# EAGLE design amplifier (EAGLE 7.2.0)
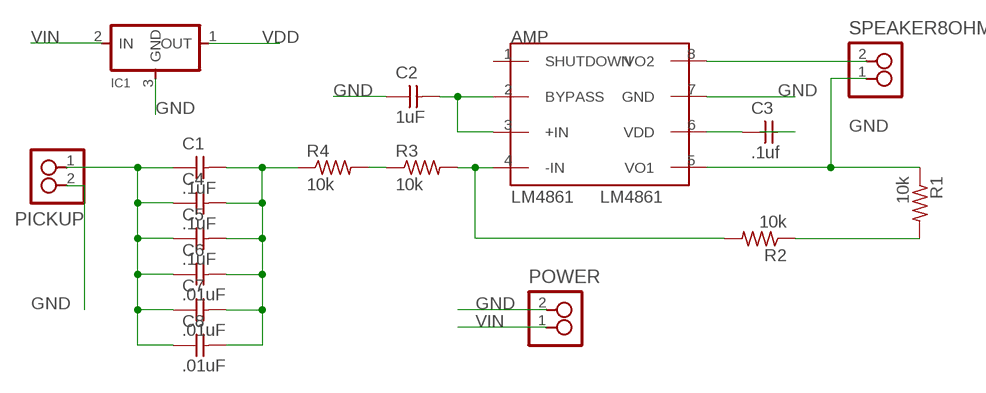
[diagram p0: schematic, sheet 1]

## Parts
AMP  LM4861  [SOIC8]
C1  .1uF  UNPOLARIZED_CAPACITOR1206  [1206]
C2  1uF  UNPOLARIZED_CAPACITOR1206  [1206]
C3  .1uf  UNPOLARIZED_CAPACITOR1206  [1206]
C4  .1uF  UNPOLARIZED_CAPACITOR1206  [1206]
C5  .1uF  UNPOLARIZED_CAPACITOR1206  [1206]
C6  .01uF  UNPOLARIZED_CAPACITOR1206  [1206]
C7  .01uF  UNPOLARIZED_CAPACITOR1206  [1206]
C8  .01uF  UNPOLARIZED_CAPACITOR1206  [1206]
IC1  REGULATORSOT23  [SOT23]
PICKUP  2_PIN_HEADERSCREW  [SCREW_2]
POWER  2_PIN_HEADERSCREW  [SCREW_2]
R1  10k  RESISTOR1206  [1206]
R2  10k  RESISTOR1206  [1206]
R3  10k  RESISTOR1206  [1206]
R4  10k  RESISTOR1206  [1206]
SPEAKER8OHM  2_PIN_HEADERSCREW  [SCREW_2]

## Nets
GND: AMP.7(GND) C2.1 C3.2 IC1.3(GND) PICKUP.2 POWER.2
N$1: AMP.4(-IN) R2.2 R3.2
N$2: R3.1 R4.2
N$3: AMP.2(BYPASS) AMP.3(+IN) C2.2
N$5: AMP.5(VO1) R1.1 SPEAKER8OHM.1
N$6: R1.2 R2.1
N$7: C1.2 C4.2 C5.2 C6.2 C7.2 C8.2 R4.1
N$9: C1.1 C4.1 C5.1 C6.1 C7.1 C8.1 PICKUP.1
SPEAKER: AMP.8(VO2) SPEAKER8OHM.2
VDD: AMP.6(VDD) C3.1 IC1.1(OUT)
VIN: IC1.2(IN) POWER.1
Unconnected: AMP.1(SHUTDOWN)

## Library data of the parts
AMP = nadya:LM4861
C1-C8 = ng:UNPOLARIZED_CAPACITOR: unpolarized_capacitor
IC1 = ng:REGULATOR
PICKUP POWER SPEAKER8OHM = ng:2_PIN_HEADER: 2 SMT pin pads
R1-R4 = ng:RESISTOR

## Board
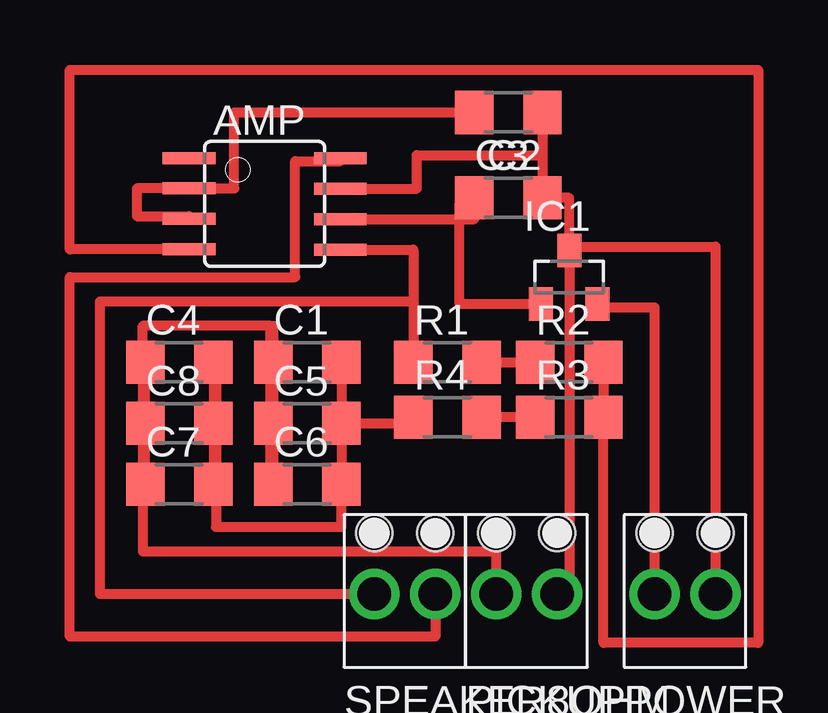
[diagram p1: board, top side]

No outline drawn. Coordinates in mm, seen from the top.
Copper layers (1*16): Top 0.035mm / dielectric 1.5mm / Bottom 0.035mm
Design rules "default": minimum track width 10mil, minimum drill 24mil, track to track 8mil, track to pad 8mil, pad to pad 8mil, via to via 8mil, smd to smd 8mil, copper to edge 40mil, drill to drill 8mil, minimum pad ring 10mil, minimum via ring 8mil, stop-mask expansion 4mil, vias tented up to drill 0mil, thermal gap 10mil

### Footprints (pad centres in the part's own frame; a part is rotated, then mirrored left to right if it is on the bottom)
SOIC8 = smd 0.5 x 2.2: 1 -1.905,-3.154; 2 -0.645,-3.154; 3 0.625,-3.154; 4 1.895,-3.154; 5 1.905,3.154; 6 0.635,3.154; 7 -0.635,3.154; 8 -1.905,3.154
1206 = smd 1.6 x 1.803: 1 -1.422,0; 2 1.422,0
SOT23 = smd 1 x 1.4: 1 -1.179,-1.125; 2 1.179,-1.125; 3 0,1.1
SCREW_2 = drill 1.4 pad 2.108: 1 -1.27,-1.27; 2 1.27,-1.27 | hole 1.5: 1.27,1.27; -1.27,1.27

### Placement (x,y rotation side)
AMP  9.4,18.8 270 top
C1  11.18,12.19 0 top
C2  19.56,22.61 180 top
C3  19.56,19.05 0 top
C4  5.84,12.19 0 top
C5  11.18,9.65 0 top
C6  11.18,7.11 0 top
C7  5.84,7.11 0 top
C8  5.84,9.65 0 top
IC1  22.1,15.75 0 top
PICKUP  20.32,3.81 0 top
POWER  26.92,3.81 0 top
R1  17.02,12.19 0 top
R2  22.1,12.19 0 top
R3  22.1,9.91 0 top
R4  17.02,9.91 0 top
SPEAKER8OHM  15.24,3.81 0 top

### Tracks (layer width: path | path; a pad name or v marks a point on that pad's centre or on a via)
GND
  Top 0.406: AMP.7 15.75,19.43 15.75,20.83 20.98,20.83 | 20.98,20.83 C3.2 22.1,19.05 22.1,17.02 | C2.1 20.98,20.83 | 22.1,17.02 IC1.3 22.1,2.79 21.59,2.79 PICKUP.2 | 22.1,17.02 28.19,17.02 POWER.2
N$1
  Top 0.406: R2.2 R3.2 23.52,0.51 29.97,0.51 29.97,24.38 1.27,24.38 1.27,16.9 AMP.4
N$2
  Top 0.406: R3.1 R4.2
N$3
  Top 0.406: AMP.3 6.24,18.29 4.06,18.29 4.06,19.44 AMP.2 8.13,19.44 8.13,22.61 C2.2
N$5
  Top 0.406: AMP.5 15.6,16.89 R1.1 15.6,14.73 2.54,14.73 2.54,2.54 SPEAKER8OHM.1
N$6
  Top 0.406: R1.2 R2.1
N$7
  Top 0.406: C5.2 C6.2 12.6,5.33 7.37,5.33 7.37,12.19 C4.2 C8.2 C7.2 | C1.2 C5.2 | C5.2 15.6,9.65 R4.1
N$9
  Top 0.406: 4.32,12.19 C4.1 C8.1 C7.1 | 4.32,12.19 4.32,13.72 9.65,13.72 | 9.65,13.72 9.75,13.72 C1.1 C5.1 C6.1 9.65,7.11 9.65,13.72 | 4.32,12.19 4.32,4.32 19.05,4.32 PICKUP.1
SPEAKER
  Top 0.406: AMP.8 12.55,20.57 10.67,20.57 10.67,15.75 1.27,15.75 1.27,0.76 16.51,0.76 SPEAKER8OHM.2
VDD
  Top 0.406: AMP.6 18.14,18.16 C3.1 18.14,18.8 17.53,18.8 17.53,14.62 IC1.1
VIN
  Top 0.406: IC1.2 23.28,14.48 25.65,14.48 POWER.1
